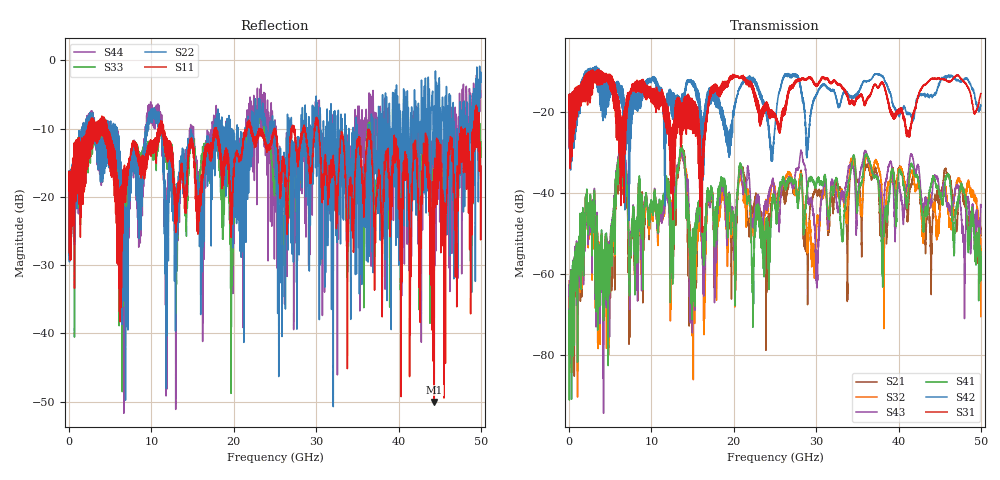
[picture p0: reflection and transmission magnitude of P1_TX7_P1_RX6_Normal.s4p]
!Keysight Technologies,N5225B,MY57041031,A.13.20.10
!Date: Friday, May 31, 2019 11:22:52
!Correction: S11(Full 4 Port(1,2,3,4))
!S12(Full 4 Port(1,2,3,4))
!S13(Full 4 Port(1,2,3,4))
!S14(Full 4 Port(1,2,3,4))
!S21(Full 4 Port(1,2,3,4))
!S22(Full 4 Port(1,2,3,4))
!S23(Full 4 Port(1,2,3,4))
!S24(Full 4 Port(1,2,3,4))
!S31(Full 4 Port(1,2,3,4))
!S32(Full 4 Port(1,2,3,4))
!S33(Full 4 Port(1,2,3,4))
!S34(Full 4 Port(1,2,3,4))
!S41(Full 4 Port(1,2,3,4))
!S42(Full 4 Port(1,2,3,4))
!S43(Full 4 Port(1,2,3,4))
!S44(Full 4 Port(1,2,3,4))
!S4P File: Measurements: <S11,S12,S13,S14>,
!<S21,S22,S23,S24>,
!<S31,S32,S33,S34>,
!<S41,S42,S43,S44>:
# Hz S  dB  R 50.0
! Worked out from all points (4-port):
!   5000 points, 10 MHz to 50 GHz, reference 50 ohm
!   strongest paths, dB at 10 MHz, 12.51 GHz, 25.01 GHz, 37.51 GHz, 50 GHz:
!     S31: -19.4, -39.6, -20.9, -14.0, -15.5
!     S42: -19.4, -15.6, -23.2, -10.9, -18.6
!     S41: -69.0, -45.6, -43.2, -37.3, -54.6
!     S43: -62.7, -45.7, -40.4, -36.5, -43.6
!     S32: -72.4, -45.2, -39.5, -32.9, -70.5
!     S21: -61.7, -45.3, -41.6, -37.3, -50.7
!   lowest |S11| = -50.0 dB at 44.34 GHz (marker M1), VSWR 1.01, Z = 50 - j0.311 ohm
!   |S11| at or under -10 dB: 4.613 GHz to 10.86 GHz (6.246 GHz wide, 80.7 % of centre); 11.46 GHz to 17.73 GHz (6.278 GHz wide, 43 % of centre); 30.28 GHz to 47.6 GHz (17.32 GHz wide, 44.5 % of centre)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
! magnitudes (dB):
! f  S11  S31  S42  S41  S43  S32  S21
! 10 MHz  -19.1  -19.4  -19.4  -69.0  -62.7  -72.4  -61.7
! 6.23 GHz  -30.7  -23.6  -16.5  -29.0  -28.5  -29.0  -29.6
! 7.41 GHz  -14.5  -15.2  -17.1  -58.3  -58.0  -55.0  -58.1
! 13.7 GHz  -15.1  -25.7  -15.8  -29.0  -30.1  -30.4  -29.4
! 14.85 GHz  -11.7  -17.1  -12.4  -60.0  -68.2  -67.3  -66.5
! 44.34 GHz  -50.0  -11.9  -15.8  -36.5  -36.3  -44.2  -42.9
! 50 GHz  -15.5  -15.5  -18.6  -54.6  -43.6  -70.5  -50.7
